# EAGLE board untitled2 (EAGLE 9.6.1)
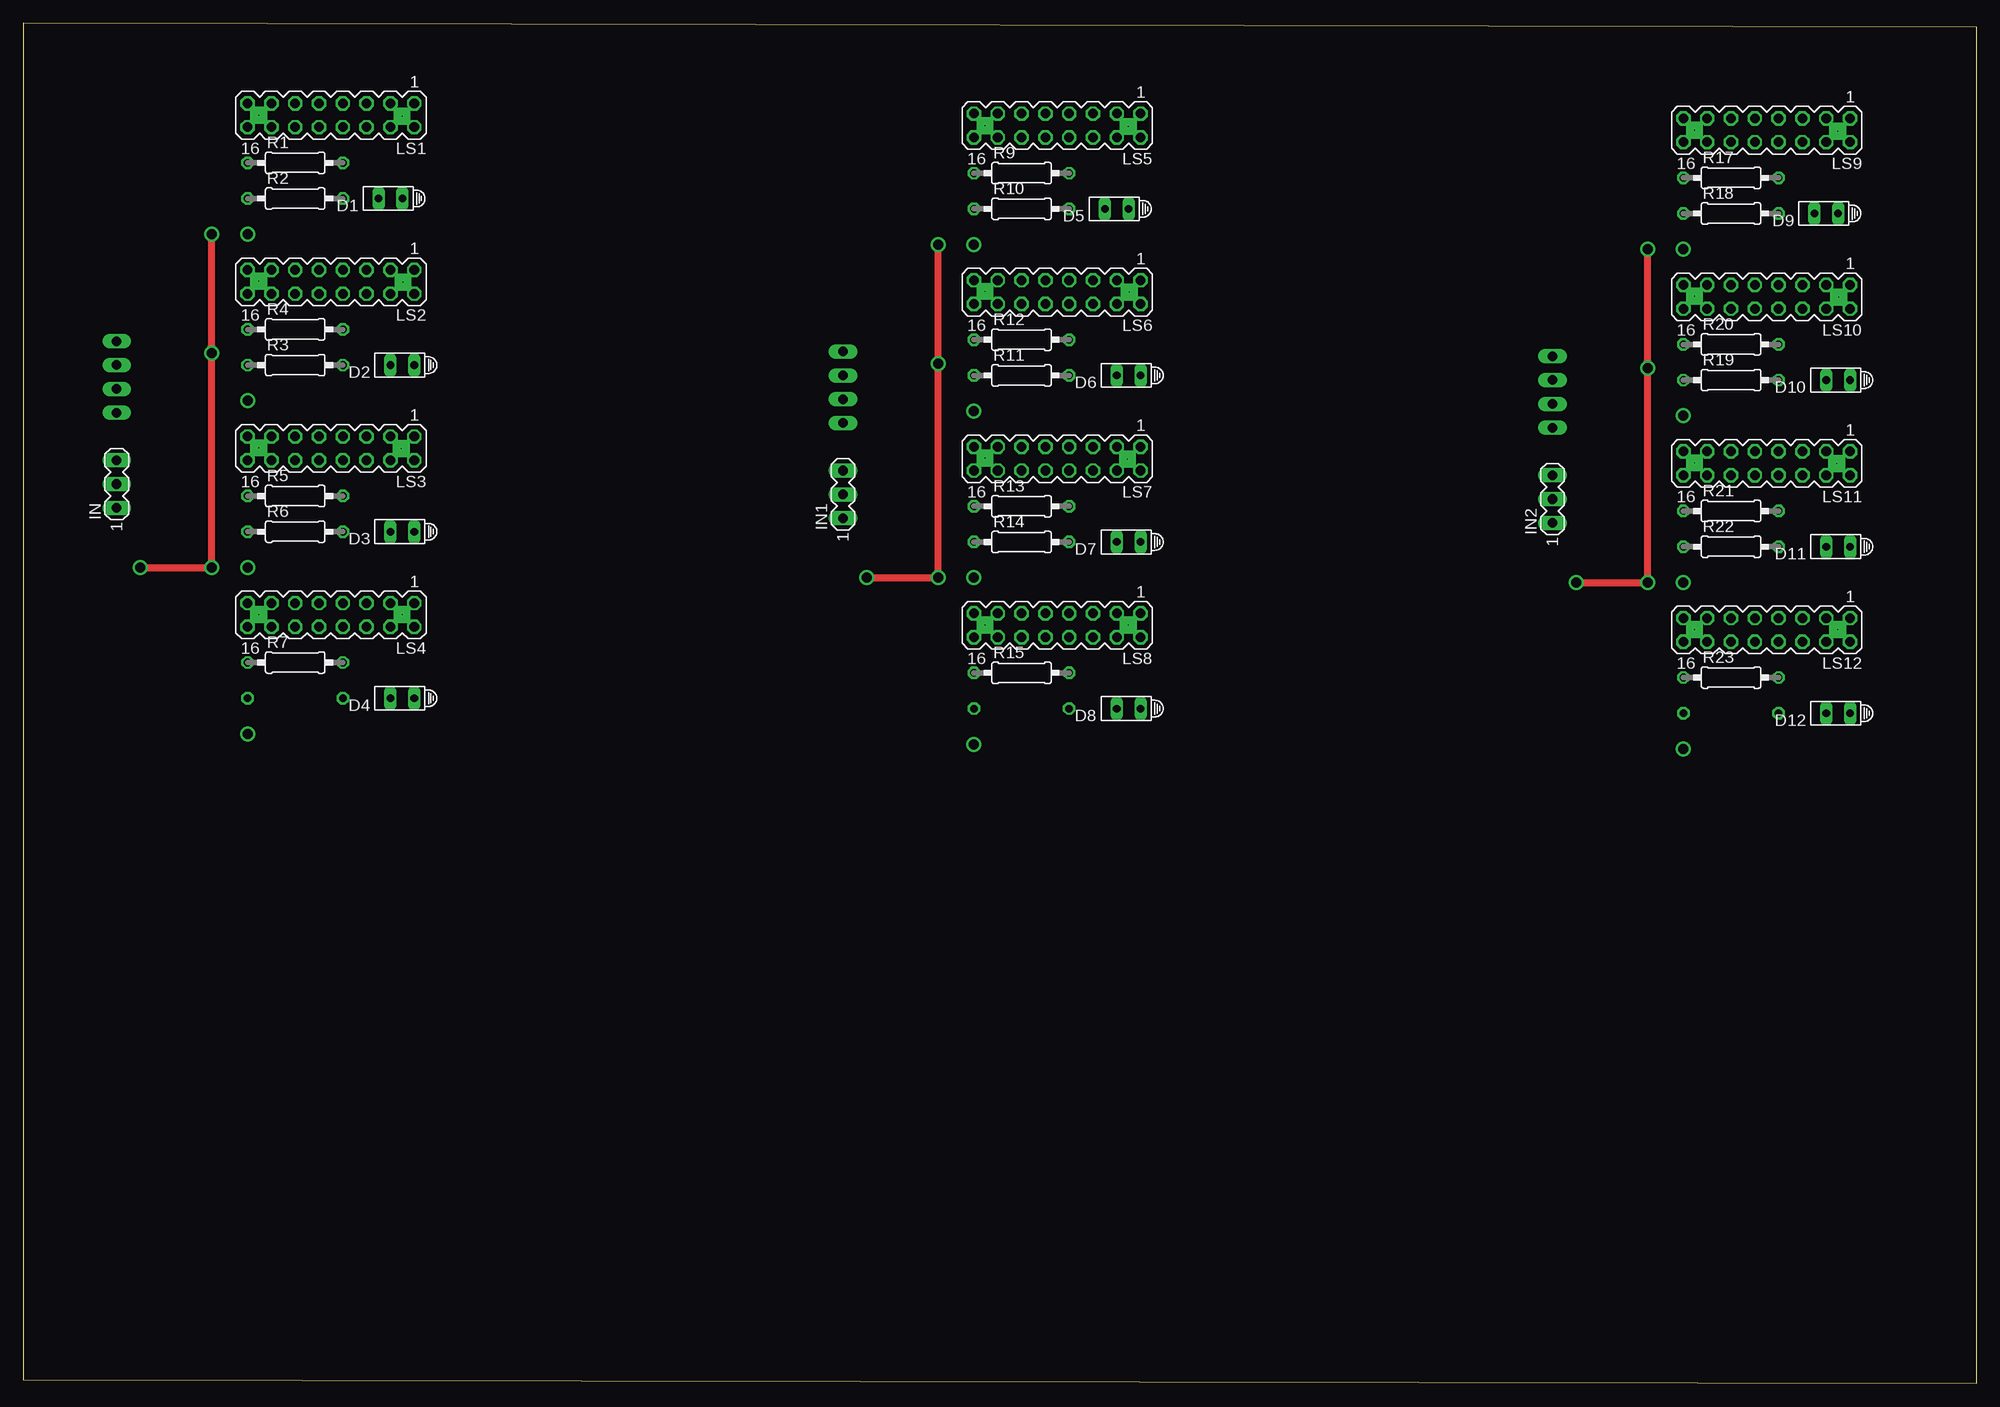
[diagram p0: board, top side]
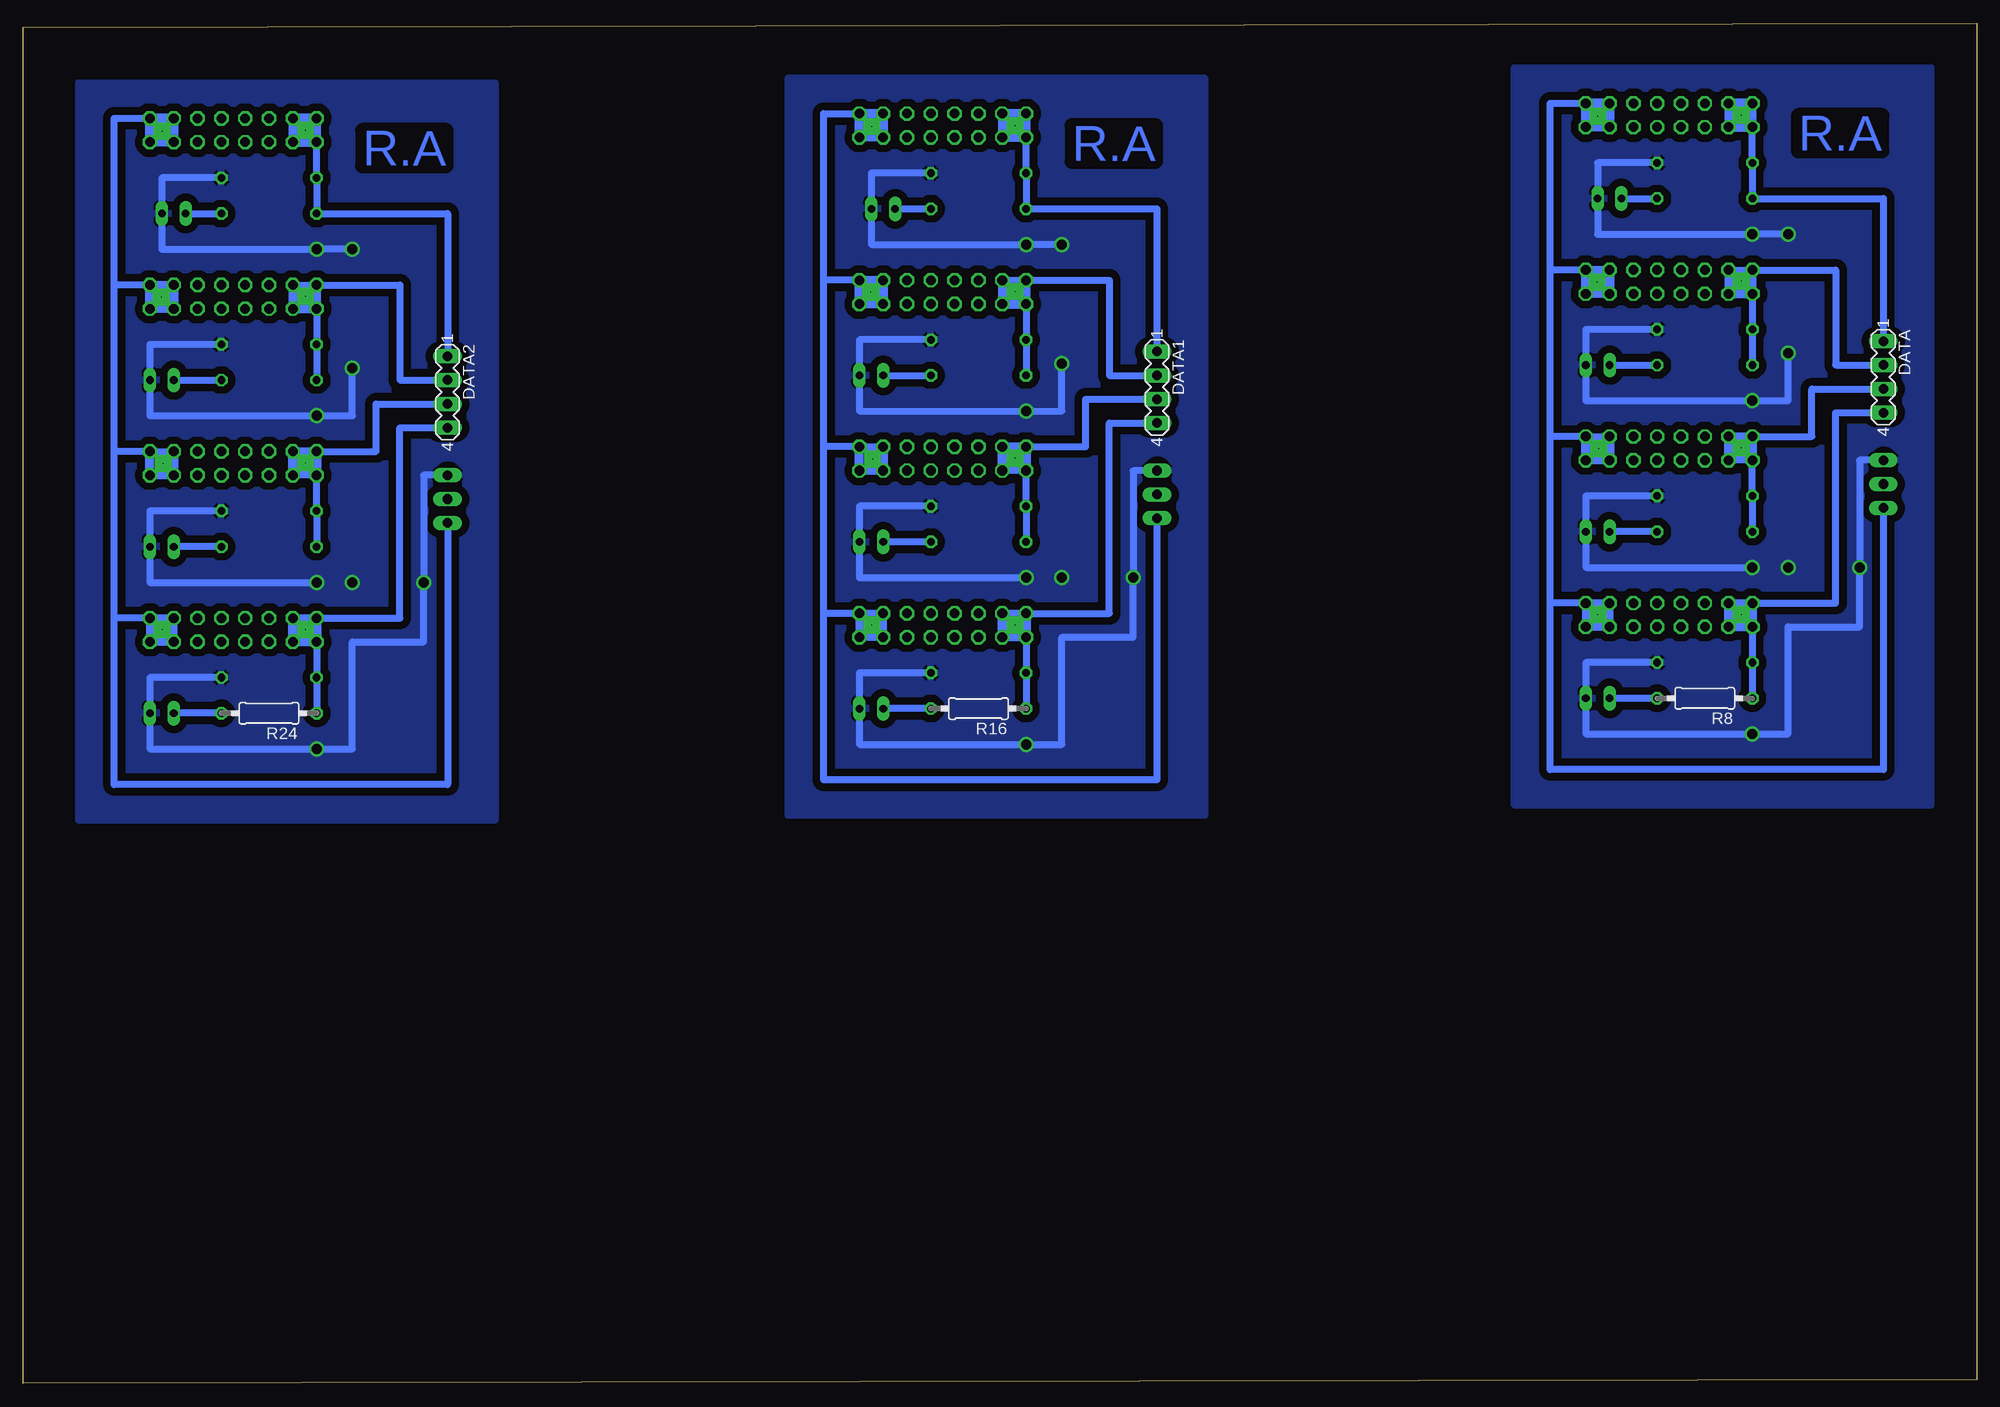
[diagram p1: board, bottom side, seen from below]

Size 208.4 x 145.17 mm. Coordinates in mm from the lower left corner, seen from the top.
Outline: 0,0.4 208.4,0 208.4,144.77 0,145.17 0,0.4
Copper layers (1*16): Top 0.035mm / dielectric 1.5mm / Bottom 0.035mm
Design rules "default": minimum track width 6mil, minimum drill 0.35mm, track to track 6mil, track to pad 6mil, pad to pad 6mil, via to via 6mil, smd to smd 6mil, copper to edge 40mil, drill to drill 6mil, minimum pad ring 10mil, minimum via ring 8mil, stop-mask expansion 4mil, vias tented up to drill 0mil, thermal gap 10mil

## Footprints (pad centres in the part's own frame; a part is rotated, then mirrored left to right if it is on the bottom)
HLMP6 = drill 0.813 long: A -1.27,0; K 1.27,0
MA04-1 = drill 1.016 long: 1 -3.81,0; 2 -1.27,0; 3 1.27,0; 4 3.81,0
MA03-1 = drill 1.016 long: 1 -2.54,0; 2 0,0; 3 2.54,0
MA08-2 = drill 1.016 octagon: 1 -8.89,-1.27; 2 -8.89,1.27; 3 -6.35,-1.27; 4 -6.35,1.27; 5 -3.81,-1.27; 6 -3.81,1.27; 7 -1.27,-1.27; 8 -1.27,1.27; 9 1.27,-1.27; 10 1.27,1.27; 11 3.81,-1.27; 12 3.81,1.27; 13 6.35,-1.27; 14 6.35,1.27; 15 8.89,-1.27; 16 8.89,1.27
0207/10 = drill 0.813 octagon: 1 -5.08,0; 2 5.08,0

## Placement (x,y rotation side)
D1  HLMP6  [HLMP6]  39.16,126.48 180 top
D2  HLMP6  [HLMP6]  40.43,108.7 180 top
D3  HLMP6  [HLMP6]  40.43,90.92 180 top
D4  HLMP6  [HLMP6]  40.43,73.14 180 top
D5  HLMP6  [HLMP6]  116.66,125.38 180 top
D6  HLMP6  [HLMP6]  117.93,107.6 180 top
D7  HLMP6  [HLMP6]  117.93,89.82 180 top
D8  HLMP6  [HLMP6]  117.93,72.04 180 top
D9  HLMP6  [HLMP6]  192.36,124.88 180 top
D10  HLMP6  [HLMP6]  193.63,107.1 180 top
D11  HLMP6  [HLMP6]  193.63,89.32 180 top
D12  HLMP6  [HLMP6]  193.63,71.54 180 top
DATA  [MA04-1]  9.95,107.43 270 bottom
DATA1  [MA04-1]  87.45,106.33 270 bottom
DATA2  [MA04-1]  163.15,105.83 270 bottom
IN  [MA03-1]  9.95,96 90 top
IN1  [MA03-1]  87.45,94.9 90 top
IN2  [MA03-1]  163.15,94.4 90 top
LS1  [MA08-2]  32.81,135.37 180 top
LS2  [MA08-2]  32.81,117.59 180 top
LS3  [MA08-2]  32.81,99.81 180 top
LS4  [MA08-2]  32.81,82.03 180 top
LS5  [MA08-2]  110.31,134.27 180 top
LS6  [MA08-2]  110.31,116.49 180 top
LS7  [MA08-2]  110.31,98.71 180 top
LS8  [MA08-2]  110.31,80.93 180 top
LS9  [MA08-2]  186.01,133.77 180 top
LS10  [MA08-2]  186.01,115.99 180 top
LS11  [MA08-2]  186.01,98.21 180 top
LS12  [MA08-2]  186.01,80.43 180 top
R1  [0207/10]  29,130.29 0 top
R2  [0207/10]  29,126.48 0 top
R3  [0207/10]  29,108.7 0 top
R4  [0207/10]  29,112.51 0 top
R5  [0207/10]  29,94.73 0 top
R6  [0207/10]  29,90.92 0 top
R7  [0207/10]  29,76.95 0 top
R8  [0207/10]  29,73.14 180 bottom
R9  [0207/10]  106.5,129.19 0 top
R10  [0207/10]  106.5,125.38 0 top
R11  [0207/10]  106.5,107.6 0 top
R12  [0207/10]  106.5,111.41 0 top
R13  [0207/10]  106.5,93.63 0 top
R14  [0207/10]  106.5,89.82 0 top
R15  [0207/10]  106.5,75.85 0 top
R16  [0207/10]  106.5,72.04 180 bottom
R17  [0207/10]  182.2,128.69 0 top
R18  [0207/10]  182.2,124.88 0 top
R19  [0207/10]  182.2,107.1 0 top
R20  [0207/10]  182.2,110.91 0 top
R21  [0207/10]  182.2,93.13 0 top
R22  [0207/10]  182.2,89.32 0 top
R23  [0207/10]  182.2,75.35 0 top
R24  [0207/10]  182.2,71.54 180 bottom

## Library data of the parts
D1-D12 = display-hp; MF: AGILENT TECHNOLOGIES; MPN: HLMP-6500; OC_FARNELL: 1652490; OC_NEWARK: 40K0088
DATA DATA1 DATA2 IN IN1 IN2 LS1-LS12 = con-lstb; OC_FARNELL: unknown; OC_NEWARK: unknown
R1-R24 = rcl; SPICEPREFIX: R

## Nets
GND: D1.A D2.A D3.A D4.A IN.3 R1.2 R4.2 R5.2 R7.2
GND1: D5.A D6.A D7.A D8.A IN1.3 R9.2 R12.2 R13.2 R15.2
GND2: D9.A D10.A D11.A D12.A IN2.3 R17.2 R20.2 R21.2 R23.2
N$1: DATA.1 LS1.13 LS1.14 LS1.15 LS1.16 R1.1 R2.1
N$2: D2.K R3.2
N$3: DATA.2 LS2.13 LS2.14 LS2.15 LS2.16 R3.1 R4.1
N$4: D3.K R6.2
N$5: D1.K R2.2
N$6: DATA.3 LS3.13 LS3.14 LS3.15 LS3.16 R5.1 R6.1
N$7: D4.K R8.2
N$8: DATA.4 LS4.13 LS4.14 LS4.15 LS4.16 R7.1 R8.1
N$9: IN.1 LS1.1 LS1.2 LS1.3 LS1.4 LS2.1 LS2.2 LS2.3 LS2.4 LS3.1 LS3.2 LS3.3 LS3.4 LS4.1 LS4.2 LS4.3 LS4.4
N$21: D5.K R10.2
N$22: DATA1.1 LS5.13 LS5.14 LS5.15 LS5.16 R9.1 R10.1
N$23: D6.K R11.2
N$24: DATA1.2 LS6.13 LS6.14 LS6.15 LS6.16 R11.1 R12.1
N$25: D7.K R14.2
N$26: DATA1.3 LS7.13 LS7.14 LS7.15 LS7.16 R13.1 R14.1
N$27: D8.K R16.2
N$28: DATA1.4 LS8.13 LS8.14 LS8.15 LS8.16 R15.1 R16.1
N$29: IN1.1 LS5.1 LS5.2 LS5.3 LS5.4 LS6.1 LS6.2 LS6.3 LS6.4 LS7.1 LS7.2 LS7.3 LS7.4 LS8.1 LS8.2 LS8.3 LS8.4
N$41: D9.K R18.2
N$42: DATA2.1 LS9.13 LS9.14 LS9.15 LS9.16 R17.1 R18.1
N$43: D10.K R19.2
N$44: DATA2.2 LS10.13 LS10.14 LS10.15 LS10.16 R19.1 R20.1
N$45: D11.K R22.2
N$46: DATA2.3 LS11.13 LS11.14 LS11.15 LS11.16 R21.1 R22.1
N$47: D12.K R24.2
N$48: DATA2.4 LS12.13 LS12.14 LS12.15 LS12.16 R23.1 R24.1
N$49: IN2.1 LS9.1 LS9.2 LS9.3 LS9.4 LS10.1 LS10.2 LS10.3 LS10.4 LS11.1 LS11.2 LS11.3 LS11.4 LS12.1 LS12.2 LS12.3 LS12.4

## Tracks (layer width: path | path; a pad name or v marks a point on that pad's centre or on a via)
GND  (via drill 0.03 pad 1.27, 0.76 pad 1.27, 1.07 pad 0.81)
  Top 0.762: v12.49,87.11 v20.11,87.11 v20.11,109.97 v20.11,122.67
  Bottom 0.762: R1.2 40.43,130.29 D1.A 40.43,122.67 v23.92,122.67 v20.11,122.67 | R4.2 41.7,112.51 D2.A 41.7,104.89 v23.92,104.89 20.11,104.89 v20.11,109.97 | R5.2 41.7,94.73 D3.A 41.7,87.11 v23.92,87.11 | R7.2 41.7,76.95 D4.A 41.7,69.33 v23.92,69.33 20.11,69.33 20.11,80.76 12.49,80.76 v12.49,87.11 12.49,98.54 IN.3
  pour Bottom (isolate 0.813): 49.32,140.45 4.87,140.45 4.87,61.71 49.32,61.71
GND1  (via drill 0.03 pad 1.27, 0.76 pad 1.27, 1.07 pad 0.81)
  Top 0.762: v89.99,86.01 v97.61,86.01 v97.61,108.87 v97.61,121.57
  Bottom 0.762: R9.2 117.93,129.19 D5.A 117.93,121.57 v101.42,121.57 v97.61,121.57 | R12.2 119.2,111.41 D6.A 119.2,103.79 v101.42,103.79 97.61,103.79 v97.61,108.87 | R13.2 119.2,93.63 D7.A 119.2,86.01 v101.42,86.01 | R15.2 119.2,75.85 D8.A 119.2,68.23 v101.42,68.23 97.61,68.23 97.61,79.66 89.99,79.66 v89.99,86.01 89.99,97.44 IN1.3
  pour Bottom (isolate 0.813): 126.82,139.35 82.37,139.35 82.37,60.61 126.82,60.61
GND2  (via drill 0.03 pad 1.27, 0.76 pad 1.27, 1.07 pad 0.81)
  Top 0.762: v165.69,85.51 v173.31,85.51 v173.31,108.37 v173.31,121.07
  Bottom 0.762: R17.2 193.63,128.69 D9.A 193.63,121.07 v177.12,121.07 v173.31,121.07 | R20.2 194.9,110.91 D10.A 194.9,103.29 v177.12,103.29 173.31,103.29 v173.31,108.37 | R21.2 194.9,93.13 D11.A 194.9,85.51 v177.12,85.51 | R23.2 194.9,75.35 D12.A 194.9,67.73 v177.12,67.73 173.31,67.73 173.31,79.16 165.69,79.16 v165.69,85.51 165.69,96.94 IN2.3
  pour Bottom (isolate 0.813): 202.52,138.85 158.07,138.85 158.07,60.11 202.52,60.11
N$1
  Bottom 0.762: LS1.16 R1.1 R2.1 9.95,126.48 DATA.1
  Bottom 0.965: LS1.15 LS1.13 LS1.14 LS1.16 LS1.15
N$2
  Bottom 0.762: D2.K R3.2
N$3
  Bottom 0.762: LS2.16 R4.1 R3.1 | DATA.2 15.03,108.7 15.03,118.86 LS2.15 LS2.13
  Bottom 0.965: LS2.13 LS2.14 LS2.16 LS2.15
N$4
  Bottom 0.762: R6.2 D3.K
N$5
  Bottom 0.762: D1.K R2.2
N$6
  Bottom 0.762: R6.1 R5.1 LS3.16 LS3.14 | LS3.15 17.57,101.08 17.57,106.16 DATA.3
  Bottom 0.965: LS3.14 LS3.13 LS3.15 LS3.16
N$7
  Bottom 0.762: R8.2 D4.K
N$8
  Bottom 0.762: LS4.13 LS4.15 15.03,83.3 15.03,103.62 DATA.4 | LS4.16 R7.1 R8.1
  Bottom 0.965: LS4.13 LS4.14 LS4.16 LS4.15
N$9
  Bottom 0.762: IN.1 9.95,65.52 45.51,65.52 45.51,83.3 | LS1.1 45.51,136.64 45.51,118.86 | 45.51,83.3 45.51,101.08 | 45.51,101.08 45.51,118.86 | LS2.1 45.51,118.86 | LS3.3 LS3.1 45.51,101.08 | 45.51,83.3 LS4.1 LS4.3
  Bottom 0.813: LS4.1 LS4.2 LS4.4 LS4.3
  Bottom 0.965: LS3.3 LS3.4 LS3.2 LS3.1 | LS2.3 LS2.4 LS2.2 LS2.1 LS2.3 | LS1.4 LS1.2 LS1.1 LS1.3 LS1.4
N$10  (via drill 0.76 pad 1.27)
  other vias: 9.9,98.57
N$11  (via drill 0.76 pad 1.27)
  other vias: 9.9,95.87
N$12  (via drill 0.76 pad 1.27)
  other vias: 9.9,93.47
N$13  (via drill 0.1 pad 1.8)
  other vias: 25.1,117.67
N$14  (via drill 0.1 pad 1.8)
  other vias: 40.5,117.57
N$15  (via drill 0.1 pad 1.8)
  other vias: 25.1,99.87
N$16  (via drill 0.1 pad 1.8)
  other vias: 40.3,99.77
N$17  (via drill 0.1 pad 1.8)
  other vias: 25.1,82.07
N$18  (via drill 0.1 pad 1.8)
  other vias: 40.4,82.07
N$19  (via drill 0.1 pad 1.8)
  other vias: 40.4,135.27
N$20  (via drill 0.1 pad 1.8)
  other vias: 25.1,135.37
N$21
  Bottom 0.762: D5.K R10.2
N$22
  Bottom 0.762: LS5.16 R9.1 R10.1 87.45,125.38 DATA1.1
  Bottom 0.965: LS5.15 LS5.13 LS5.14 LS5.16 LS5.15
N$23
  Bottom 0.762: D6.K R11.2
N$24
  Bottom 0.762: LS6.16 R12.1 R11.1 | DATA1.2 92.53,107.6 92.53,117.76 LS6.15 LS6.13
  Bottom 0.965: LS6.13 LS6.14 LS6.16 LS6.15
N$25
  Bottom 0.762: R14.2 D7.K
N$26
  Bottom 0.762: R14.1 R13.1 LS7.16 LS7.14 | LS7.15 95.07,99.98 95.07,105.06 DATA1.3
  Bottom 0.965: LS7.14 LS7.13 LS7.15 LS7.16
N$27
  Bottom 0.762: R16.2 D8.K
N$28
  Bottom 0.762: LS8.13 LS8.15 92.53,82.2 92.53,102.52 DATA1.4 | LS8.16 R15.1 R16.1
  Bottom 0.965: LS8.13 LS8.14 LS8.16 LS8.15
N$29
  Bottom 0.762: IN1.1 87.45,64.42 123.01,64.42 123.01,82.2 | LS5.1 123.01,135.54 123.01,117.76 | 123.01,82.2 123.01,99.98 | 123.01,99.98 123.01,117.76 | LS6.1 123.01,117.76 | LS7.3 LS7.1 123.01,99.98 | 123.01,82.2 LS8.1 LS8.3
  Bottom 0.813: LS8.1 LS8.2 LS8.4 LS8.3
  Bottom 0.965: LS7.3 LS7.4 LS7.2 LS7.1 | LS6.3 LS6.4 LS6.2 LS6.1 LS6.3 | LS5.4 LS5.2 LS5.1 LS5.3 LS5.4
N$30  (via drill 0.76 pad 1.27)
  other vias: 87.4,97.47
N$31  (via drill 0.76 pad 1.27)
  other vias: 87.4,94.77
N$32  (via drill 0.76 pad 1.27)
  other vias: 87.4,92.37
N$33  (via drill 0.1 pad 1.8)
  other vias: 102.6,116.57
N$34  (via drill 0.1 pad 1.8)
  other vias: 118,116.47
N$35  (via drill 0.1 pad 1.8)
  other vias: 102.6,98.77
N$36  (via drill 0.1 pad 1.8)
  other vias: 117.8,98.67
N$37  (via drill 0.1 pad 1.8)
  other vias: 102.6,80.97
N$38  (via drill 0.1 pad 1.8)
  other vias: 117.9,80.97
N$39  (via drill 0.1 pad 1.8)
  other vias: 117.9,134.17
N$40  (via drill 0.1 pad 1.8)
  other vias: 102.6,134.27
N$41
  Bottom 0.762: D9.K R18.2
N$42
  Bottom 0.762: LS9.16 R17.1 R18.1 163.15,124.88 DATA2.1
  Bottom 0.965: LS9.15 LS9.13 LS9.14 LS9.16 LS9.15
N$43
  Bottom 0.762: D10.K R19.2
N$44
  Bottom 0.762: LS10.16 R20.1 R19.1 | DATA2.2 168.23,107.1 168.23,117.26 LS10.15 LS10.13
  Bottom 0.965: LS10.13 LS10.14 LS10.16 LS10.15
N$45
  Bottom 0.762: R22.2 D11.K
N$46
  Bottom 0.762: R22.1 R21.1 LS11.16 LS11.14 | LS11.15 170.77,99.48 170.77,104.56 DATA2.3
  Bottom 0.965: LS11.14 LS11.13 LS11.15 LS11.16
N$47
  Bottom 0.762: R24.2 D12.K
N$48
  Bottom 0.762: LS12.13 LS12.15 168.23,81.7 168.23,102.02 DATA2.4 | LS12.16 R23.1 R24.1
  Bottom 0.965: LS12.13 LS12.14 LS12.16 LS12.15
N$49
  Bottom 0.762: IN2.1 163.15,63.92 198.71,63.92 198.71,81.7 | LS9.1 198.71,135.04 198.71,117.26 | 198.71,81.7 198.71,99.48 | 198.71,99.48 198.71,117.26 | LS10.1 198.71,117.26 | LS11.3 LS11.1 198.71,99.48 | 198.71,81.7 LS12.1 LS12.3
  Bottom 0.813: LS12.1 LS12.2 LS12.4 LS12.3
  Bottom 0.965: LS11.3 LS11.4 LS11.2 LS11.1 | LS10.3 LS10.4 LS10.2 LS10.1 LS10.3 | LS9.4 LS9.2 LS9.1 LS9.3 LS9.4
N$50  (via drill 0.76 pad 1.27)
  other vias: 163.1,96.97
N$51  (via drill 0.76 pad 1.27)
  other vias: 163.1,94.27
N$52  (via drill 0.76 pad 1.27)
  other vias: 163.1,91.87
N$53  (via drill 0.1 pad 1.8)
  other vias: 178.3,116.07
N$54  (via drill 0.1 pad 1.8)
  other vias: 193.7,115.97
N$55  (via drill 0.1 pad 1.8)
  other vias: 178.3,98.27
N$56  (via drill 0.1 pad 1.8)
  other vias: 193.5,98.17
N$57  (via drill 0.1 pad 1.8)
  other vias: 178.3,80.47
N$58  (via drill 0.1 pad 1.8)
  other vias: 193.6,80.47
N$59  (via drill 0.1 pad 1.8)
  other vias: 193.6,133.67
N$60  (via drill 0.1 pad 1.8)
  other vias: 178.3,133.77

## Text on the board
Bottom: R.A | R.A | R.A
